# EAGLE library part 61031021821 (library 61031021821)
Headers & Wire Housings WR-PHD Header 2.54mm SMT Source: Datasheet
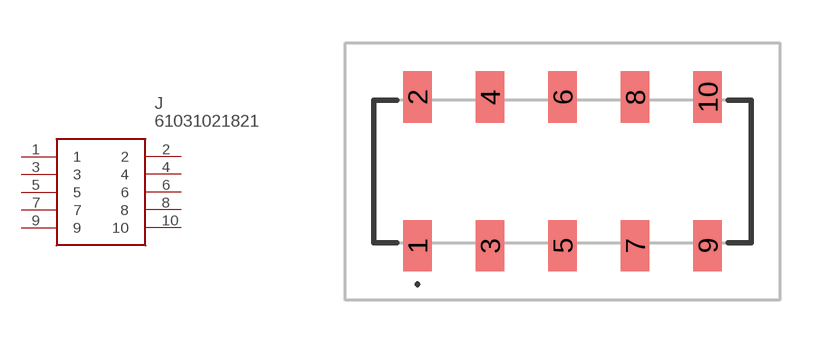
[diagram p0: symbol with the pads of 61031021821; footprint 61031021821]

Designator prefix J

## 61031021821 (Description: Headers & Wire Housings WR-PHD Header 2.54mm SMT; Height: 7.75mm; Manufacturer_Name: Wurth Elektronik; Manufacturer_Part_Number: 61031021821; Mouser_Part_Number: 710-61031021821; Mouser_Price-Stock: https://www.mouser.co.uk/ProductDetail/Wurth-Elektronik/61031021821?qs=Cb2nCFKsA8qcYgZIDjCpgw%3D%3D)  [61031021821]
1  1
2  2
3  3
4  4
5  5
6  6
7  7
8  8
9  9
10  10

## Footprint 61031021821 (pad centres in mm)
61031021821-1
smd 1 x 1.8: 1 -5.08,-2.6; 2 -5.08,2.6; 3 -2.54,-2.6; 4 -2.54,2.6; 5 0,-2.6; 6 0,2.6; 7 2.54,-2.6; 8 2.54,2.6; 9 5.08,-2.6; 10 5.08,2.6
